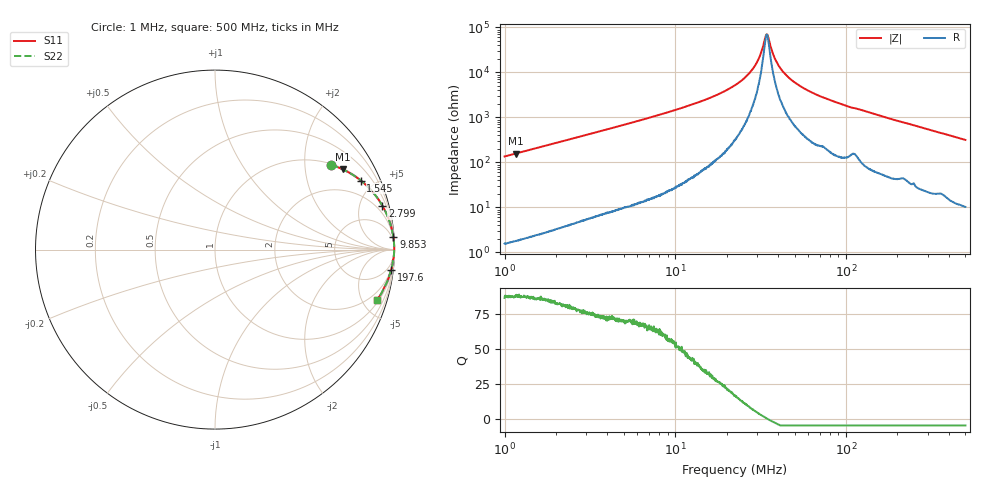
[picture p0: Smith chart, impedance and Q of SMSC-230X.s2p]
!s-Parameter Generated by FASTRON Sdn. Bhd.
!FASTRON P/N : SMSC-230X
!Keysight Technologies,E4991B,MY54100416,A.01.15
!Date: Thu Mar 19 15:03:25 2026
!Version  : Rev00 Thu Mar 19 15:03:25 2026
!Data & Calibration Information:
!PortZ  Port1:50+j0  Port2:50+j0
!When reading, reference impedance value at option line is always used.
!Remarks : This data is being provided solely for informational purposes.
!Freq	S11	S21	S12	S22
# Hz S dB R 50
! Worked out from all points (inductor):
!   1601 points, 1 MHz to 500 MHz, reference 50 ohm
!   read as one part in series: L = 21.6 uH near 1.032 MHz
!   highest Q = 88 at 1.159 MHz (marker M1), where L = 21.6 uH
!   self-resonance near 34.28 MHz
!   S11 on the Smith chart (normalised r, x): 1 MHz: 1.03, +2.72; 1.545 MHz: 1.05, +4.20; 2.799 MHz: 1.10, +7.61; 9.853 MHz: 2, +29; 197.6 MHz: 2, -17; 500 MHz: 1.21, -6.33
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1000000  -1.93 36.1  -4.59 -53.2  -4.59 -53.2  -1.93 36.1
1159046  -1.51 32.2  -5.46 -57.1  -5.46 -57.1  -1.51 32.2
1544998  -0.93 25.3  -7.37 -64.0  -7.37 -64.0  -0.93 25.3
2799090  -0.32 14.7  -11.93 -74.6  -11.93 -74.6  -0.32 14.7
2820919  -0.31 14.6  -11.99 -74.7  -11.99 -74.7  -0.31 14.6
7957584  -0.05 5.0  -21.11 -84.0  -21.11 -84.0  -0.05 5.0
9852770  -0.03 4.0  -23.21 -85.0  -23.21 -85.0  -0.03 4.0
1.60732e7  -0.02 2.1  -28.83 -86.1  -28.83 -86.1  -0.02 2.1
2.236068e7  -0.01 1.1  -34.32 -85.4  -34.32 -85.4  -0.01 1.1
2.889466e7  -0.01 0.4  -42.34 -79.8  -42.34 -79.8  -0.01 0.4
3.09871e7  -0.01 0.3  -46.73 -73.1  -46.73 -73.1  -0.01 0.3
3.349022e7  -0.01 0.1  -54.86 -38.1  -54.86 -38.1  -0.01 0.1
3.441328e7  -0.01 -0.0  -56.80 2.8  -56.80 2.8  -0.01 -0.0
3.522469e7  -0.01 -0.1  -54.77 37.0  -54.77 37.0  -0.01 -0.1
3.851633e7  -0.01 -0.3  -45.81 72.7  -45.81 72.7  -0.01 -0.3
4.2444e7  -0.01 -0.5  -40.60 79.5  -40.60 79.5  -0.01 -0.5
4.957817e7  -0.02 -0.9  -35.80 82.8  -35.80 82.8  -0.02 -0.9
6.307767e7  -0.02 -1.6  -31.12 84.0  -31.12 84.0  -0.02 -1.6
1.017089e8  -0.05 -3.2  -25.00 82.6  -25.00 82.6  -0.05 -3.2
1.77937e8  -0.09 -5.9  -19.71 81.3  -19.71 81.3  -0.09 -5.9
1.976111e8  -0.11 -6.6  -18.72 80.5  -18.72 80.5  -0.11 -6.6
5e8  -0.49 -17.3  -10.51 70.8  -10.51 70.8  -0.49 -17.3
